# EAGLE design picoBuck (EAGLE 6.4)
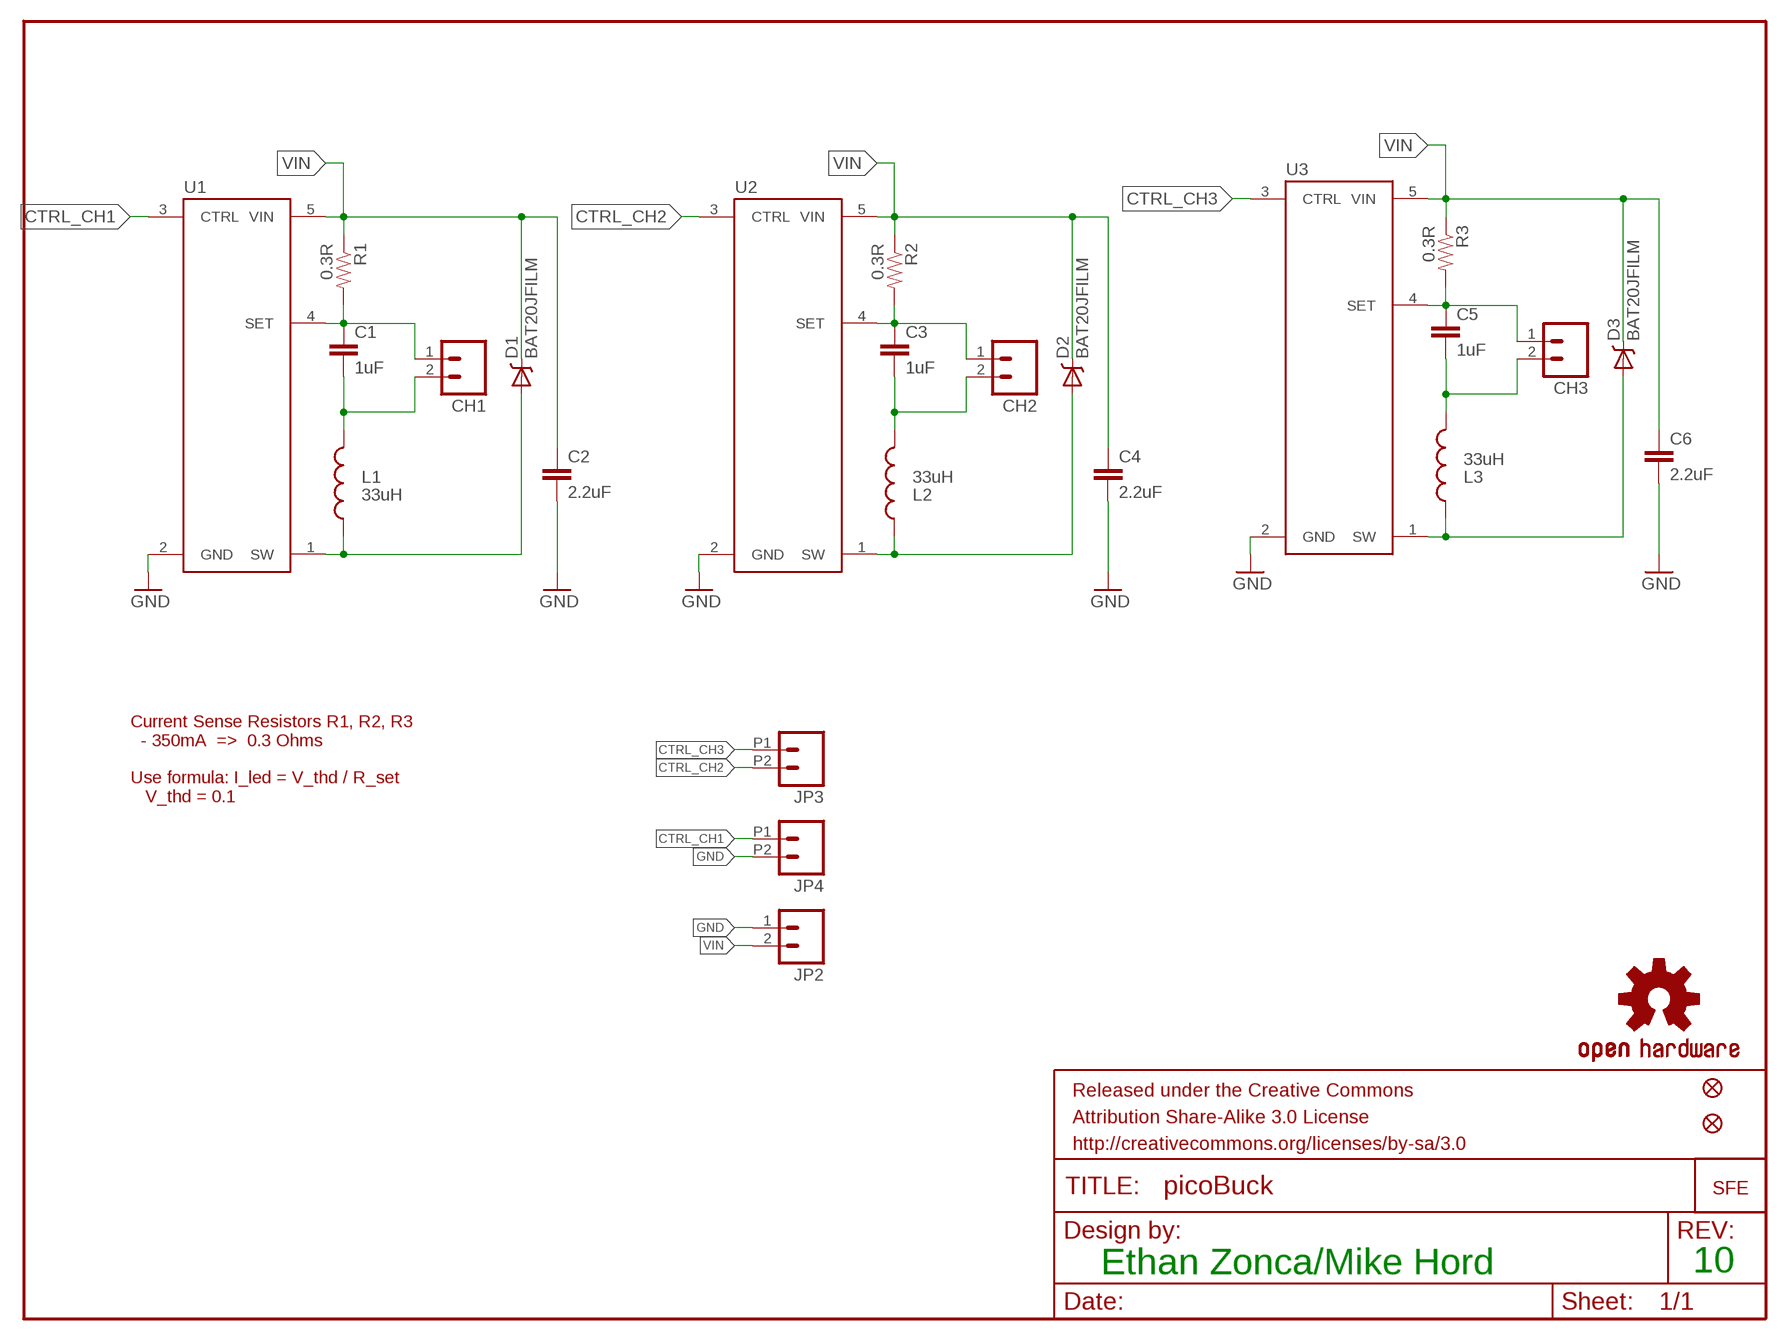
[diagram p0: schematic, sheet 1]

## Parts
C1  1uF  1.0UF-25V-+80/-20(0805)  [0805]
C2  2.2uF  2.2UF-25V-+80/-20(0805)  [0805]
C3  1uF  1.0UF-25V-+80/-20(0805)  [0805]
C4  2.2uF  2.2UF-25V-+80/-20(0805)  [0805]
C5  1uF  1.0UF-25V-+80/-20(0805)  [0805]
C6  2.2uF  2.2UF-25V-+80/-20(0805)  [0805]
CH1  M023.5MM_LOCK  [SCREWTERMINAL-3.5MM-2_LOCK]
CH2  M023.5MM_LOCK  [SCREWTERMINAL-3.5MM-2_LOCK]
CH3  M023.5MM_LOCK  [SCREWTERMINAL-3.5MM-2_LOCK]
D1  BAT20JFILM  [SOD-323]
D2  BAT20JFILM  [SOD-323]
D3  BAT20JFILM  [SOD-323]
FID1  FIDUCIALUFIDUCIAL  [MICRO-FIDUCIAL]
FID2  FIDUCIALUFIDUCIAL  [MICRO-FIDUCIAL]
FRAME1  FRAME-LETTER  [CREATIVE_COMMONS]
JP2  M023.5MM_LOCK  [SCREWTERMINAL-3.5MM-2_LOCK]
JP3  M022.54MM_SCREWTERM  [1X02_2.54_SCREWTERM]
JP4  M022.54MM_SCREWTERM  [1X02_2.54_SCREWTERM]
L1  33uH  INDUCTORBOURNS_SRN6045  [SRN6045]
L2  33uH  INDUCTORBOURNS_SRN6045  [SRN6045]
L3  33uH  INDUCTORBOURNS_SRN6045  [SRN6045]
LOGO1  OSHW-LOGOS  [OSHW-LOGO-S]
LOGO2  LOGO-SFENEW  [SFE-NEW-WEBLOGO]
R1  0.3R  0.3OHM-1/8W-1%(0805)  [0805]
R2  0.3R  0.3OHM-1/8W-1%(0805)  [0805]
R3  0.3R  0.3OHM-1/8W-1%(0805)  [0805]
U1  AL8805  [SOT23-5]
U2  AL8805  [SOT23-5]
U3  AL8805  [SOT23-5]

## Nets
CTRL_CH1: JP4.P1 U1.3(CTRL)
CTRL_CH2: JP3.P2 U2.3(CTRL)
CTRL_CH3: JP3.P1 U3.3(CTRL)
GND: C2.2 C4.2 C6.2 JP2.1 JP4.P2 U1.2(GND) U2.2(GND) U3.2(GND)
IND1-1: D1.2(A) L1.1 U1.1(SW)
IND2-1: D2.2(A) L2.1 U2.1(SW)
IND3-1: D3.2(A) L3.1 U3.1(SW)
N$5 [power]: C1.2 CH1.2 L1.2
N$9 [power]: C3.2 CH2.2 L2.2
N$11: C1.1 CH1.1 R1.2 U1.4(SET)
N$13: C3.1 CH2.1 R2.2 U2.4(SET)
N$16 [power]: C5.2 CH3.2 L3.2
N$18: C5.1 CH3.1 R3.2 U3.4(SET)
VIN: C2.1 C4.1 C6.1 D1.1(C) D2.1(C) D3.1(C) JP2.2 R1.1 R2.1 R3.1 U1.5(VIN) U2.5(VIN) U3.5(VIN)

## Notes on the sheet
- Current Sense Resistors R1, R2, R3
    - 350mA  =>  0.3 Ohms
  
  Use formula: I_led = V_thd / R_set
     V_thd = 0.1
- Ethan Zonca/Mike Hord | 10

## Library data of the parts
C1 C3 C5 = SparkFun-Capacitors:1.0UF-25V-+80/-20(0805); PROD_ID: CAP-11625; VALUE: 1.0uF
C2 C4 C6 = SparkFun-Capacitors:2.2UF-25V-+80/-20(0805); PROD_ID: CAP-11624
CH1-CH3 JP2 = SparkFun:M02: Header 2
D1-D3 = SparkFun-DiscreteSemi:BAT20JFILM: 23V, 1A Schottky diode, SOD-323 package; PROD_ID: DIO-11623
FID1 FID2 = SparkFun-Aesthetics:FIDUCIAL: Fiducial Alignment Points
FRAME1 = SparkFun-Aesthetics:FRAME-LETTER: Schematic Frame
JP3 JP4 = SparkFun-Connectors:M02: Standard 2-pin 0.1" header. Use with
L1-L3 = SparkFun-Passives:INDUCTOR: Inductors; PROD_ID: NDUC-11627
LOGO1 = SparkFun-Aesthetics:OSHW-LOGO: Open Source Hardware Logo This logo indicates the piece of hardware it is found on incorporates a OSHW license and/or adheres to the definition of open source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
LOGO2 = SparkFun-Aesthetics:LOGO-SFE: Spark Fun Electronics PCB Logo
R1-R3 = SparkFun-Resistors:0.3OHM-1/8W-1%(0805); PROD_ID: RES-11622; VALUE: 0.3
U1-U3 = SparkFun-PowerIC:AL8805: Constant current LED driver PWM-able 1MHz switch freq 6V-36V Up to 1A LED current; PROD_ID: IC-11626; VALUE: AL8805WS

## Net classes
0 default: width 0.254 mm
1 power: width 0.508 mm

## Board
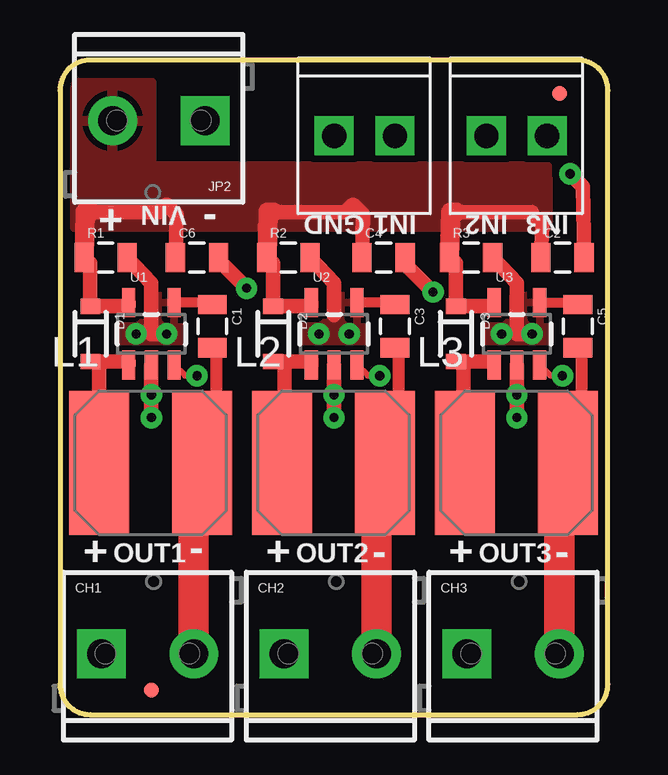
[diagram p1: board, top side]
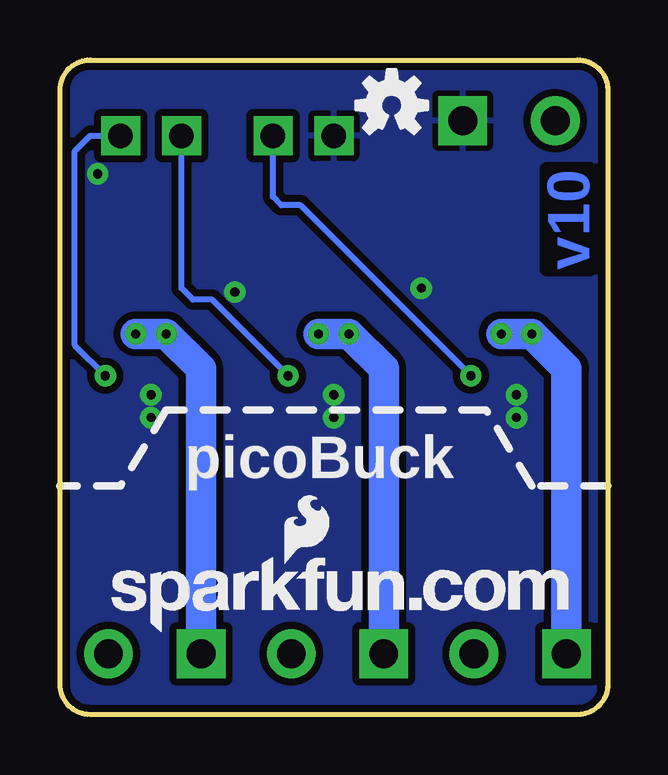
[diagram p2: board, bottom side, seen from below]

Size 22.85 x 27.3 mm. Coordinates in mm from the lower left corner, seen from the top.
Outline: 0,26.02 0,1.27 arc90 1.27,0 21.58,0 arc90 22.85,1.27 22.85,26.02 arc90 21.58,27.3 1.27,27.3 arc90 0,26.02
Copper layers (1*16): Top 0.035mm / dielectric 1.5mm / Bottom 0.035mm
Design rules "Sparkfun": minimum track width 8mil, minimum drill 20mil, track to track 8mil, track to pad 8mil, pad to pad 8mil, via to via 8mil, smd to smd 8mil, copper to edge 8mil, drill to drill 8mil, minimum pad ring 12mil, minimum via ring 10mil, stop-mask expansion 4mil, vias tented up to drill 20mil, thermal gap 10mil

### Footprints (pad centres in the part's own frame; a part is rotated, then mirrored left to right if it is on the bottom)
0805 = smd 0.8 x 1.2: 1 -0.9,0; 2 0.9,0
SCREWTERMINAL-3.5MM-2_LOCK = drill 1.2 pad 2.032 square: 1 -0.178,0 | drill 1.2 pad 2.032: 2 3.678,0
SOD-323 = smd 0.63 x 0.83: 1 -1.15,0; 2 1.15,0
MICRO-FIDUCIAL = smd 0.635 x 0.635: 1 0,0
1X02_2.54_SCREWTERM = drill 1.016 square: P1 2.54,0; P2 0,0
SRN6045 = smd 2.5 x 6: 1 -2.175,-0.175; 2 2.125,-0.175
SOT23-5 = smd 0.55 x 1.2: 1 -0.95,-1.3; 2 0,-1.3; 3 0.95,-1.3; 4 0.95,1.3; 5 -0.95,1.3

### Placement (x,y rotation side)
C1  6.35,16.19 270 top
C2  20.95,19.05 0 top
C3  13.97,16.19 270 top
C4  13.49,19.05 0 top
C5  21.59,16.19 270 top
C6  5.71,19.05 0 top
CH1  1.91,2.54 0 top
CH2  9.53,2.54 0 top
CH3  17.14,2.54 0 top
D1  1.27,15.88 270 top
D2  8.89,15.88 270 top
D3  16.51,15.88 270 top
FID1  3.81,1.02 0 top
FID2  20.83,25.91 0 top
FRAME1  not placed on the board
JP2  5.87,24.77 180 top
JP3  17.78,24.13 0 top
JP4  11.43,24.13 0 top
L1  3.81,10.67 0 top
L2  11.43,10.67 0 top
L3  19.05,10.67 0 top
LOGO1  9.02,25.4 0 bottom
LOGO2  20.7,3.43 0 bottom
R1  1.91,19.05 0 top
R2  9.53,19.05 0 top
R3  17.14,19.05 0 top
U1  3.81,15.88 0 top
U2  11.43,15.88 0 top
U3  19.05,15.88 0 top

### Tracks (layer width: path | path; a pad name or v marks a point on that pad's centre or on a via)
CTRL_CH1  (via drill 0.38 pad 0.61)
  Top 0.254: U1.3 5.22,14.13 v5.71,14.13
  Bottom 0.254: v5.71,14.13 12.82,21.24 13.62,21.24 13.97,21.59 JP4.P1
CTRL_CH2  (via drill 0.38)
  Top 0.254: U2.3 12.84,14.13 v13.34,14.13
  Bottom 0.254: v13.34,14.13 16.5,17.3 17.3,17.3 17.78,17.78 JP3.P2
CTRL_CH3  (via drill 0.38)
  Top 0.254: U3.3 20.46,14.13 v20.95,14.13
  Bottom 0.254: v20.95,14.13 22.23,15.4 22.23,23.5 21.59,24.13 JP3.P1
GND  (via drill 0.38)
  Top 0.61: U1.2 v3.81,12.38 | U2.2 v11.43,12.38 | U3.2 v19.05,12.38 | C4.2 14.34,18.84 v15.56,17.62 | C6.2 6.57,18.99 v7.78,17.78 | C2.2 21.8,22.01 v21.27,22.54
  other vias: 3.81,13.34 11.43,13.34 19.05,13.34
  pour Bottom (isolate 0.305): 0.03,27.28 22.86,27.3 22.86,0.13 0,0
IND1-1
  Top 0.61: 2.67,14.78 U1.1 2.86,14.72 D1.2 1.64,14.72 L1.1
IND2-1
  Top 0.61: 10.48,14.78 U2.1 10.48,14.72 9.37,14.72 | L2.1 9.37,10.62 9.37,14.72 | D2.2 9.37,14.72
IND3-1
  Top 0.61: 18.1,14.78 U3.1 18.1,14.72 16.83,14.72 | D3.2 16.83,14.72 | L3.1 16.83,10.62 16.83,14.72
N$5
  Top 0.508: 6.51,15.18 6.51,10.79
  Top 0.61: C1.2 6.51,15.18 | 6.51,10.79 6.33,10.62 L1.2
  Top 1.27: CH1.2 5.58,10.62 L1.2
N$9
  Top 0.508: 14.13,11.19 14.13,15.08
  Top 0.61: 14.13,11.19 L2.2 | 14.13,15.08 13.97,15.24 C3.2
  Top 1.27: CH2.2 13.2,10.62 L2.2
N$11  (via drill 0.38)
  Top 0.406: C1.1 6.22,17.18 U1.4
  Top 0.61: R1.2 3.81,18 3.81,15.88 v4.45,15.88
  Bottom 1.27: v4.45,15.88 v3.17,15.88 1.73,14.43 CH1.1
  pour Top (isolate 0.102): 2.54,15.56 5.08,15.56 5.08,17.46 3.65,17.46 3.65,16.35 2.54,16.35
N$13  (via drill 0.38)
  Top 0.406: C3.1 13.84,17.18 U2.4
  Top 0.61: R2.2 11.43,18 11.43,16.67
  Bottom 1.27: CH2.1 9.35,14.43 v10.79,15.88 v12.06,15.88
  pour Top (isolate 0.102): 10.16,15.56 12.7,15.56 12.7,17.46 11.27,17.46 11.27,16.35 10.16,16.35
N$16
  Top 0.508: 21.75,15.34 21.75,10.93
  Top 0.61: C5.2 21.75,15.34 | 21.75,10.93 21.44,10.62 L3.2
  Top 1.27: CH3.2 20.82,10.62 L3.2
N$18  (via drill 0.38, 0.38 pad 0.61)
  Top 0.406: U3.4 21.46,17.18 C5.1
  Top 0.61: R3.2 19.05,18 19.05,15.88 v19.68,15.88
  Bottom 1.27: CH3.1 16.97,14.43 v18.41,15.88 v19.68,15.88
  pour Top (isolate 0.102): 17.78,15.56 20.32,15.56 20.32,17.46 18.89,17.46 18.89,16.35 17.78,16.35
VIN
  Top 0.61: 1.27,20.95 4.13,20.95 4.45,21.27 4.87,20.85 C6.1 | R1.1 1.27,18.84 D1.1 2.86,17.02 U1.5 | R2.1 8.89,18.84 D2.1 10.48,17.02 U2.5 | 8.89,20.95 11.91,20.95 12.22,21.27 12.64,20.85 C4.1 | R3.1 16.51,18.84 D3.1 18.1,17.02 U3.5 | 16.51,20.95 19.68,20.95 19.63,20.9 20.11,20.42 C2.1
  Top 0.813: R2.1 8.68,20.95 8.89,20.95 | R3.1 16.3,20.95 16.51,20.95 | R1.1 1.05,20.95 1.27,20.95
  pour Top (isolate 0.305): 0.64,26.35 3.81,26.35 3.81,22.86 20.32,22.86 20.32,20.32 0.64,20.32

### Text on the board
Bottom: v10
tPlace: + | VIN | - | GND | IN1 | IN2 | IN3 | + | OUT1 | - | + | OUT2 | - | + | OUT3 | -
bPlace: picoBuck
